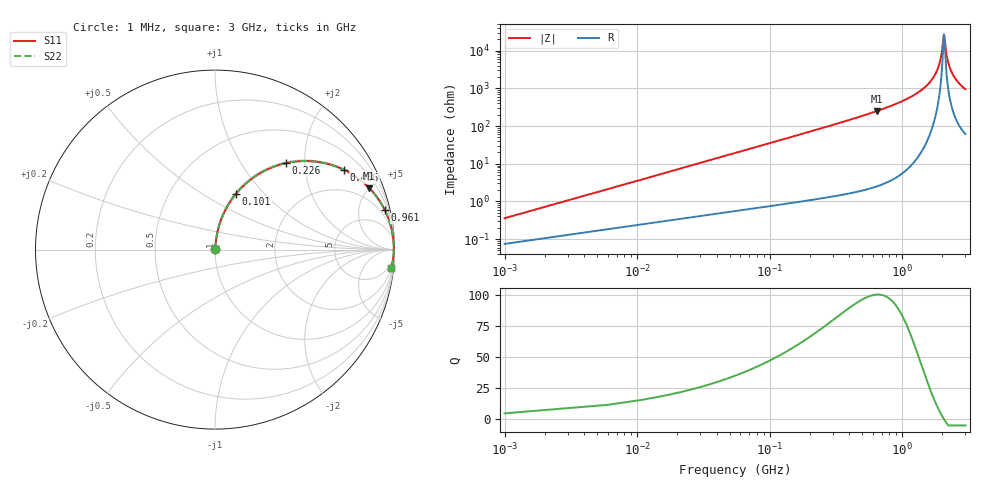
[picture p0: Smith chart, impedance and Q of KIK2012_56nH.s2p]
!version-2
!date-01.2022
!Series
# MHz S RI R 50
!Freq ReS11 ImS11 ReS21 ImS21 ReS12 ImS12 ReS22 ImS22
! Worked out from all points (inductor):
!   601 points, 1 MHz to 3 GHz, reference 50 ohm
!   read as one part in series: L = 56 nH near 16 MHz
!   highest Q = 100 at 641 MHz (marker M1), where L = 62 nH
!   self-resonance near 2.066 GHz
!   S11 on the Smith chart (normalised r, x): 1 MHz: 1.00, +0.01; 101 MHz: 1.02, +0.71; 226 MHz: 1.02, +1.61; 436 MHz: 1.03, +3.21; 961 MHz: 1.10, +8.62; 3 GHz: 2, -19
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1  0.000759 0.00351  0.9992 -0.00351  0.9992 -0.00351  0.000759 0.00351
21  0.00879 0.073  0.9912 -0.073  0.9912 -0.073  0.00879 0.073
31  0.0158 0.1069  0.9842 -0.1069  0.9842 -0.1069  0.0158 0.1069
61  0.0492 0.2031  0.9508 -0.2031  0.9508 -0.2031  0.0492 0.2031
101  0.1178 0.3119  0.8822 -0.3119  0.8822 -0.3119  0.1178 0.3119
226  0.3946 0.4817  0.6054 -0.4817  0.6054 -0.4817  0.3946 0.4817
436  0.7184 0.4444  0.2816 -0.4444  0.2816 -0.4444  0.7184 0.4444
501  0.7758 0.4119  0.2242 -0.4119  0.2242 -0.4119  0.7758 0.4119
641  0.8591 0.3429  0.1409 -0.3429  0.1409 -0.3429  0.8591 0.3429
961  0.9467 0.2189  0.0533 -0.2189  0.0533 -0.2189  0.9467 0.2189
1001  0.9526 0.2065  0.0474 -0.2065  0.0474 -0.2065  0.9526 0.2065
1501  0.9895 0.0884  0.0105 -0.0884  0.0105 -0.0884  0.9895 0.0884
1831  0.9957 0.0333  0.00426 -0.0333  0.00426 -0.0333  0.9957 0.0333
1931  0.9963 0.0188  0.00371 -0.0188  0.00371 -0.0188  0.9963 0.0188
2001  0.9964 0.00903  0.00359 -0.00903  0.00359 -0.00903  0.9964 0.00903
2051  0.9964 0.00229  0.00364 -0.00229  0.00364 -0.00229  0.9964 0.00229
2071  0.9963 -0.000353  0.00368 0.000353  0.00368 0.000353  0.9963 -0.000353
2151  0.996 -0.0107  0.004 0.0107  0.004 0.0107  0.996 -0.0107
2221  0.9956 -0.0194  0.00445 0.0194  0.00445 0.0194  0.9956 -0.0194
2336  0.9945 -0.0332  0.00551 0.0332  0.00551 0.0332  0.9945 -0.0332
2501  0.9924 -0.0518  0.00762 0.0518  0.00762 0.0518  0.9924 -0.0518
3000  0.9827 -0.102  0.0173 0.102  0.0173 0.102  0.9827 -0.102
